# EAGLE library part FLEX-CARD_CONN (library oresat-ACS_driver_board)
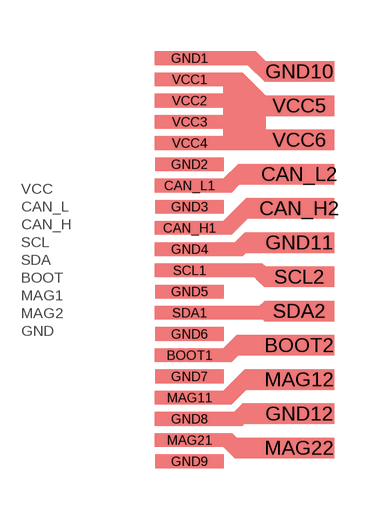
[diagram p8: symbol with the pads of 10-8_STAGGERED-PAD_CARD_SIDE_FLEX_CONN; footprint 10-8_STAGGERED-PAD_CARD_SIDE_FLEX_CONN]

Designator prefix -

## FLEX-CARD_CONN  [10-8_STAGGERED-PAD_CARD_SIDE_FLEX_CONN]
BOOT1  BOOT
BOOT2  BOOT
CAN_H1  CAN_H
CAN_H2  CAN_H
CAN_L1  CAN_L
CAN_L2  CAN_L
GND1  GND
GND2  GND
GND3  GND
GND4  GND
GND5  GND
GND6  GND
GND7  GND
GND8  GND
GND9  GND
GND10  GND
GND11  GND
GND12  GND
MAG11  MAG1
MAG12  MAG1
MAG21  MAG2
MAG22  MAG2
SCL1  SCL
SCL2  SCL
SDA1  SDA
SDA2  SDA
VCC1  VCC
VCC2  VCC
VCC3  VCC
VCC4  VCC
VCC5  VCC
VCC6  VCC

## Footprint 10-8_STAGGERED-PAD_CARD_SIDE_FLEX_CONN (pad centres in mm)
smd 2 x 0.4: BOOT1 -0.7,-2.79; CAN_H1 -0.7,0.93; CAN_L1 -0.7,2.17; GND1 -0.7,5.89; GND2 -0.7,2.79; GND3 -0.7,1.55; GND4 -0.7,0.31; GND5 -0.7,-0.93; GND6 -0.7,-2.17; GND7 -0.7,-3.41; GND8 -0.7,-4.65; GND9 -0.7,-5.89; MAG11 -0.7,-4.03; MAG21 -0.7,-5.27; SCL1 -0.7,-0.31; SDA1 -0.7,-1.55; VCC1 -0.7,5.27; VCC2 -0.7,4.65; VCC3 -0.7,4.03; VCC4 -0.7,3.41
smd 2 x 0.6: BOOT2 2.5,-2.5; CAN_H2 2.5,1.5; CAN_L2 2.5,2.5; GND10 2.5,5.5; GND11 2.5,0.5; GND12 2.5,-4.5; MAG12 2.5,-3.5; MAG22 2.5,-5.5; SCL2 2.5,-0.5; SDA2 2.5,-1.5; VCC5 2.5,4.5; VCC6 2.5,3.5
